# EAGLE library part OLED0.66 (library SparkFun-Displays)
Micro OLED TODO: Add description SparkFun Products: Micro OLED Breakout
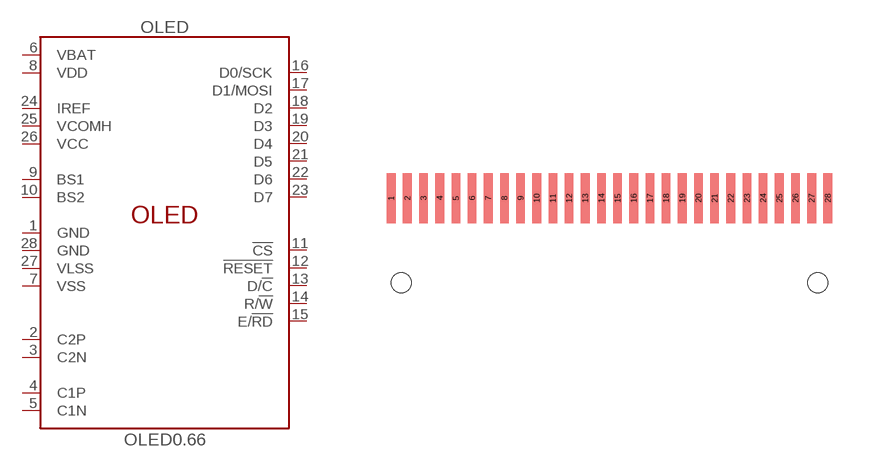
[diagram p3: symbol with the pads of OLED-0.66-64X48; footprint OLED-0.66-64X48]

Designator prefix OLED

## OLED0.66 (PROD_ID: LCD-12019)  [OLED-0.66-64X48]
1  GND
2  C2P
3  C2N
4  C1P
5  C1N
6  VBAT
7  VSS
8  VDD
9  BS1
10  BS2
11  !CS!
12  !RESET!
13  D/!C!
14  R/!W!
15  E/!RD!
16  D0/SCK
17  D1/MOSI
18  D2
19  D3
20  D4
21  D5
22  D6
23  D7
24  IREF
25  VCOMH
26  VCC
27  VLSS
28  GND

## Footprint OLED-0.66-64X48 (pad centres in mm)
OLDE display, 0.66 inch For MicroView. Specifications: Pin count: 28 Pin pitch: Area: Datasheet referenced for footprint: Example device(s): Microview breakout
smd 0.35 x 2: 1 0,0; 2 0.65,0; 3 1.3,0; 4 1.95,0; 5 2.6,0; 6 3.25,0; 7 3.9,0; 8 4.55,0; 9 5.2,0; 10 5.85,0; 11 6.5,0; 12 7.15,0; 13 7.8,0; 14 8.45,0; 15 9.1,0; 16 9.75,0; 17 10.4,0; 18 11.05,0; 19 11.7,0; 20 12.35,0; 21 13,0; 22 13.65,0; 23 14.3,0; 24 14.95,0; 25 15.6,0; 26 16.25,0; 27 16.9,0; 28 17.55,0
hole 0.8 at 17.15,-3.4
hole 0.8 at 0.4,-3.4

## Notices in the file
Licensing: Creative Commons ShareAlike 4.0 International - https://creativecommons.org/licenses/by-sa/4.0
